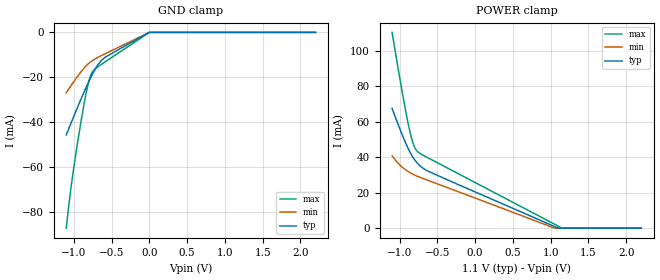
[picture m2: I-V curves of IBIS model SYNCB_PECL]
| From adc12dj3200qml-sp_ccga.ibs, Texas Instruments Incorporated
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[Model]   SYNCB_PECL
Model_type   Input
Vinl = 0.33   | Vinl & Vinh are referred to a 1.1V supply, and are an IBIS required field.
Vinh = 0.77   | However, please note that this is a differential input.
|   typ   min   max
C_comp   1.32p   1.25p   1.43p
[Voltage Range]   1.1   1.05   1.15
[Temperature Range]   25   125   -40
[Power Clamp Reference]   1.1   1.05   1.15
[GND Clamp Reference]   0   0   0
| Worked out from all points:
|   GND clamp passes 1 mA (typ) near -0.05 V on its own axis
[GND Clamp]
|   Voltage   I(typ)   I(min)   I(max)
-1.1V     -45.57mA   -26.83mA   -87.01mA
-1.037V   -40.31mA   -23.69mA   -68.88mA
-1.001V   -37.34mA   -21.93mA   -60.17mA
-911.9mV  -30.2mA    -17.84mA   -40.97mA
-852.5mV  -25.62mA   -15.45mA   -29.54mA
-816.2mV  -22.92mA   -14.2mA    -23.64mA
-783.2mV  -20.57mA   -13.24mA   -19.65mA
-753.5mV  -18.56mA   -12.52mA   -17.52mA
-713.9mV  -16.12mA   -11.7mA    -16.07mA
-581.9mV  -10.99mA   -9.451mA   -13.02mA
-1.1mV    -20.6uA    -17.89uA   -24.94uA
2.2V      0A         0A         0A
[POWER Clamp]
|   Voltage   I(typ)   I(min)   I(max)
-1.1V     67.44mA    40.75mA    110.3mA
-984.5mV  54.51mA    35.05mA    81.12mA
-918.5mV  47.78mA    32.79mA    65.61mA
-875.6mV  43.87mA    31.57mA    56.56mA
-839.3mV  41mA       30.68mA    50.16mA
-803mV    38.6mA     29.91mA    45.67mA
-773.3mV  36.97mA    29.35mA    43.58mA
-730.4mV  35.07mA    28.61mA    42.04mA
-644.6mV  32.45mA    27.22mA    40.04mA
1.048V    961.6uA    27.54uA    2.275mA
1.147V    0A         0A         60.07uA
2.2V      0A         0A         0A
